PROGRAM SerialCom
VAR
	Prefix				: BYTE:=16#F0;
	Suffix				: BYTE:=16#0F;
	fbSendData			: SendData;	
	fbReceiveData		: ReceiveData;	
	
	DataSend			: SerialComData;
	DataReceive			: SerialComData;
	DataReceiveChecked	: SerialComData;
	
	Timer				: TON;
	Send_TRIG			: R_TRIG;	
	StartSend			: BOOL;
	TestData			: LREAL;
	InvalidDataCount	: INT;
	eSendErrorID		: ComError_t ;
	SendErrCount		: INT;
	eReceiveErrorID		: ComError_t;
	ReceiveErrCount		: INT;
END_VAR

// 定时发送数据
Timer(IN:=NOT Timer.Q , PT:=T#200MS , Q=> , ET=> );
Send_TRIG(CLK:=StartSend AND Timer.Q , Q=> );
IF NOT StartSend THEN
	TestData:=0;
END_IF
IF Send_TRIG.Q THEN
	TestData:=TestData+0.1;
	DataSend.FrameHeader:=16#F0;
	DataSend.Data1:=SIN(TestData)*10000+10000;
	DataSend.Data2:=SIN(TestData+Pi/4)*5000;
	DataSend.Data3:=SIN(TestData+Pi)*10000-10000;
	DataSend.CRC:=F_DATA_TO_CRC16_CCITT(pData:=ADR(DataSend) , cbData:=SIZEOF(DataSend)-3 , crc:=16#0000 );
	DataSend.FrameEnd:=16#0F;
END_IF

IF Send_TRIG.Q OR fbSendData.Busy THEN
	fbSendData(
		pSendData:=ADR(DataSend) , 
		Length:=SIZEOF(DataSend) , 
		Busy=> , 
		Error=> , 
		TXbuffer:=TxBuffer );
END_IF
IF fbSendData.Error <> COMERROR_NOERROR THEN
	eSendErrorID := fbSendData.Error;
	SendErrCount:=SendErrCount+1;	
END_IF

fbReceiveData(
	pPrefix:=ADR(Prefix) , 
	LenPrefix:=UINT_TO_BYTE(SIZEOF(Prefix)) , 
	pSuffix:=ADR(Suffix) , 
	LenSuffix:=UINT_TO_BYTE(SIZEOF(Suffix)) , 
	pReceiveData:=ADR(DataReceive) , 
	SizeReceiveData:=SIZEOF(DataReceive) , 
	Timeout:= , 
	Reset:= , 
	DataReceived=> , 
	busy=> , 
	Error=> , 
	RxTimeout=> , 
	LenReceiveData=> , 
	RXbuffer:=RxBuffer );
IF fbReceiveData.Error <> COMERROR_NOERROR THEN
	eReceiveErrorID:=fbReceiveData.Error;
	ReceiveErrCount:=ReceiveErrCount+1;	
END_IF

// 对接收到的数据进行CRC校验，校验通过的数据有效
IF fbReceiveData.DataReceived THEN
	IF DataReceive.CRC=F_DATA_TO_CRC16_CCITT(pData:=ADR(DataReceive) , cbData:=SIZEOF(DataReceive)-3 , crc:=16#0000 ) THEN
		MEMCPY(destAddr:=ADR(DataReceiveChecked) , srcAddr:=ADR(DataReceive)  , n:=SIZEOF(DataReceive) );
	ELSE
		InvalidDataCount:=InvalidDataCount+1;
	END_IF
END_IF

END_PROGRAM
